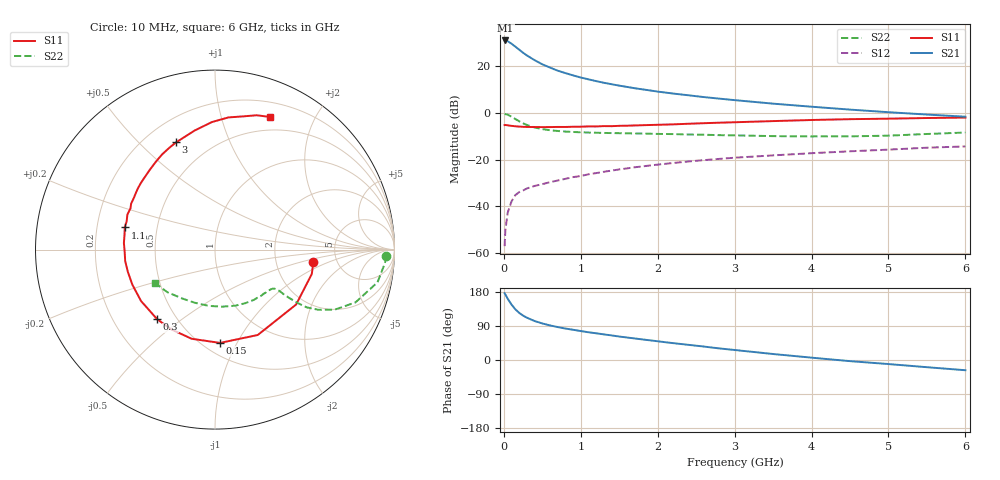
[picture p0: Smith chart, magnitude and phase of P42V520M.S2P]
! SIEMENS Small Signal Semiconductors
! BFP182
! Si NPN RF Bipolar Junction Transistor in SOT143
! VCE = 2.5 V  IC = 20 mA
! Common Emitter S-Parameters:  March  1996
# GHz  S  MA  R  50
!  f  S11  S21  S12  S22
! GHz  MAG  ANG  MAG  ANG  MAG  ANG  MAG  ANG
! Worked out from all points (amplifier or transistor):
!   36 points, 10 MHz to 6 GHz, reference 50 ohm
!   highest |S21| = 31.1 dB at 20 MHz (marker M1)
!   |S21| within 3 dB of that: start of sweep to 162.9 MHz
!   unconditionally stable (mu >= 1): 689.1 MHz to 5.413 GHz
!   at 250 MHz: K = 0.53, MSG = 29.5 dB, |S12| = -33.2 dB
!   at 1.4 GHz: K = 1.21, MAG = 15.7 dB, |S12| = -24.7 dB
!   at 6 GHz: K = 0.95, MSG = 6.4 dB, |S12| = -14.3 dB
!   S11 on the Smith chart (normalised r, x): 10 MHz: 3.33, -0.65; 150 MHz: 0.60, -0.86; 300 MHz: 0.39, -0.41; 1.1 GHz: 0.32, +0.11; 3 GHz: 0.32, +0.65; 6 GHz: 0.35, +1.44
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0.01  0.5528 -7.0  35.95 176.2  0.0014 84.7  0.9557 -2.1
0.02  0.5561 -14.2  36.07 172.8  0.0031 85.2  0.9496 -4.6
0.05  0.5458 -34.1  34.77 161.7  0.0073 79.5  0.9235 -11.4
0.1  0.5321 -63.4  30.69 146.1  0.0128 63.9  0.8361 -20.6
0.15  0.5206 -86.9  26.54 133.6  0.0175 59.5  0.7454 -26.7
0.2  0.5136 -104.7  22.85 124.3  0.0202 53.8  0.6666 -30.2
0.25  0.5067 -118.6  19.64 117.1  0.0219 51.7  0.6043 -32.2
0.3  0.5043 -129.7  17.21 111.6  0.0242 49.9  0.5547 -32.8
0.4  0.5019 -145.2  13.62 102.8  0.0274 49.8  0.4917 -33.1
0.5  0.5002 -157.0  11.12 96.5  0.0299 49.7  0.4531 -33.0
0.6  0.5011 -165.7  9.456 91.3  0.033 50.9  0.4294 -32.7
0.7  0.5044 -172.8  8.117 86.9  0.0358 52.1  0.413 -32.8
0.8  0.5036 -179.1  7.194 83.0  0.0389 52.6  0.4015 -33.1
1  0.5107 170.8  5.785 76.4  0.0447 54.2  0.387 -34.3
1.1  0.5177 166.2  5.289 73.2  0.0487 53.7  0.3824 -35.3
1.5  0.5328 151.3  3.878 61.9  0.0619 53.8  0.3705 -40.2
2.2  0.5729 129.7  2.625 44.5  0.085 49.9  0.3543 -52.3
3  0.6357 109.9  1.896 26.4  0.1104 43.5  0.3326 -69.9
3.5  0.6731 99.7  1.593 15.8  0.1238 39.0  0.3205 -82.6
4.5  0.7403 84.2  1.187 -3.0  0.1515 30.5  0.3168 -110.8
5.5  0.7835 72.8  0.93 -19.0  0.181 22.2  0.3562 -138.3
6  0.8004 67.4  0.836 -27.0  0.1928 17.1  0.3828 -151.0
